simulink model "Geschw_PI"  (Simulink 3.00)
settings: Solver=ode5  SolverMode=SingleTasking  StartTime=0.0  StopTime=0.4  RelTol=1e-3  AbsTol=1e-6
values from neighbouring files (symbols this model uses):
  bm = 4    [PI_Par.m]    (also in Red_Par.m)
  K_St = 1/FD_Stern    (= 2.27848101266)    [PI_Par.m]    (also in Red_Par.m = 1/FD_Stern)
  KP = (1/K_St)*(2*d*T_St-T)/T    (= 23.3767988889)    [PI_Par.m]
  qA = 0    [PI_Par.m]    (also in Red_Par.m)
  T_St = M_Stern/FD_Stern    (= 2.82860759494)    [PI_Par.m]    (also in Red_Par.m = M_Stern/FD_Stern)
  tb = vm/bm    (= 0.5)    [PI_Par.m]    (also in Red_Par.m)
  te = tv+tb    (= 1.2853981634)    [PI_Par.m]    (also in Red_Par.m)
  TN = T*(2*d-T/T_St)    (= 0.0693971006366)    [PI_Par.m]
  tv = se/vm    (= 0.785398163397)    [PI_Par.m]    (also in Red_Par.m)
  Vorz = 1    [PI_Par.m]    (also in Red_Par.m)
  z0 = (1/KM)*(rh)    (= 1.25)    [PI_Par.m]    (also in Red_Par.m = (1/KM)*(rh))

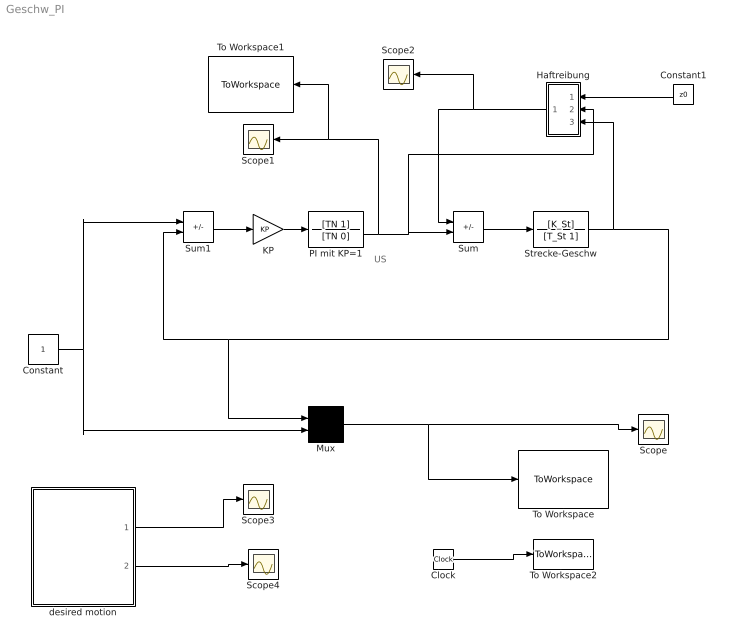
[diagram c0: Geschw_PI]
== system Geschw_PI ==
  note: US
  Clock : Clock
  Constant : Constant  Value=1
  Constant1 : Constant  Orientation=left  Value=z0
  Haftreibung : Subsystem  Orientation=left
  KP : Gain  Gain=KP  SaturateOnIntegerOverflow=on
  Mux : Mux  Inputs=2
  PI mit KP=1 : TransferFcn  Numerator=[TN 1]  Denominator=[TN 0]
  Scope{,1..4} (5 alike) : Scope
  Strecke-Geschw : TransferFcn  Numerator=[K_St]  Denominator=[T_St 1]
  Sum : Sum  Inputs=-+  SaturateOnIntegerOverflow=on
  Sum1 : Sum  Inputs=+-  SaturateOnIntegerOverflow=on
  To Workspace : ToWorkspace  VariableName=PI_MMin_SP  SampleTime=0.001  SaveFormat=Matrix
  To Workspace1 : ToWorkspace  VariableName=PI_MMin_US_SP  SampleTime=0.001  SaveFormat=Matrix
  To Workspace2 : ToWorkspace  VariableName=Zeit_SP  SampleTime=0.001  SaveFormat=Matrix
  desired motion : Subsystem
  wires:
  Sum1/1 -> KP/1
  KP/1 -> PI mit KP=1/1
  PI mit KP=1/1 -> Sum/2, Haftreibung/2(US), Scope1/1, To Workspace1/1
  Strecke-Geschw/1 -> Sum1/2, Mux/1, Haftreibung/3(qp)
  Sum/1 -> Strecke-Geschw/1
  Constant1/1 -> Haftreibung/1(z0)
  Haftreibung/1(Out1) -> Sum/1, Scope2/1
  Mux/1 -> Scope/1, To Workspace/1
  Clock/1 -> To Workspace2/1
  desired motion/1(qd) -> Scope3/1
  desired motion/2(vd) -> Scope4/1
  Constant/1 -> Mux/2, Sum1/1

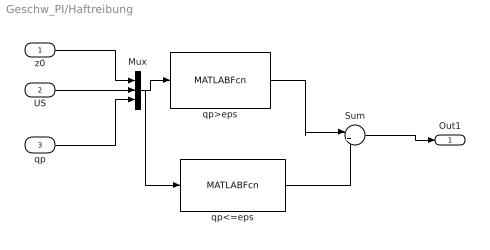
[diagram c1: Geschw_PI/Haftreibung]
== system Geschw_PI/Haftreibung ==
  z0 : Inport  Port=1  PortWidth=-1  SampleTime=-1  DataType=auto
  US : Inport  Port=2  PortWidth=-1  SampleTime=-1  DataType=auto
  qp : Inport  Port=3  PortWidth=-1  SampleTime=-1  DataType=auto
  Mux : Mux  Inputs=3
  Sum : Sum  Inputs=|++  SaturateOnIntegerOverflow=on
  qp<=eps : MATLABFcn  MATLABFcn=(abs(u(3)) < eps) *min(abs(u(2)),u(1))* sign(u(2))*sign(u(1))  OutputWidth=1  OutputSignalType=auto
  qp>eps : MATLABFcn  MATLABFcn=(abs(u(3)) > eps) * sign(u(3))*u(1)  OutputWidth=1  OutputSignalType=auto
  Out1 : Outport  Port=1  InitialOutput=0
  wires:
  z0/1 -> Mux/1
  US/1 -> Mux/2
  qp/1 -> Mux/3
  Mux/1 -> qp>eps/1, qp<=eps/1
  Sum/1 -> Out1/1
  qp>eps/1 -> Sum/1
  qp<=eps/1 -> Sum/2

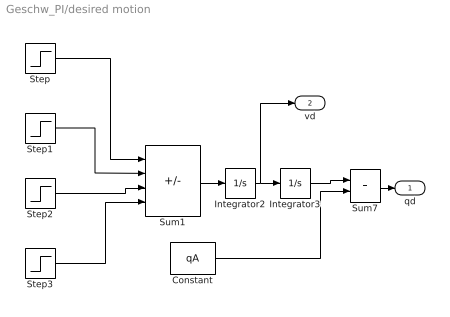
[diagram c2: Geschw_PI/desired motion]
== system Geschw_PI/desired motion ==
  Constant : Constant  Value=qA
  Integrator2 : Integrator  ExternalReset=none  InitialConditionSource=internal  InitialCondition=0  LimitOutput=off  UpperSaturationLimit=inf  LowerSaturationLimit=-inf  ShowSaturationPort=off  ShowStatePort=off  AbsoluteTolerance=auto
  Integrator3 : Integrator  ExternalReset=none  InitialConditionSource=internal  InitialCondition=0  LimitOutput=off  UpperSaturationLimit=inf  LowerSaturationLimit=-inf  ShowSaturationPort=off  ShowStatePort=off  AbsoluteTolerance=auto
  Step : Step  Time=0  Before=0  After=bm*Vorz  SampleTime=0.005
  Step1 : Step  Time=tb  Before=0  After=bm*Vorz  SampleTime=0.005
  Step2 : Step  Time=tv  Before=0  After=bm*Vorz  SampleTime=0.005
  Step3 : Step  Time=te  Before=0  After=bm*Vorz  SampleTime=0.005
  Sum1 : Sum  Inputs=+--+  SaturateOnIntegerOverflow=on
  Sum7 : Sum  Inputs=++  SaturateOnIntegerOverflow=on
  qd : Outport  Port=1  InitialOutput=0
  vd : Outport  Port=2
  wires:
  Step/1 -> Sum1/1
  Step1/1 -> Sum1/2
  Step2/1 -> Sum1/3
  Step3/1 -> Sum1/4
  Sum1/1 -> Integrator2/1
  Integrator2/1 -> Integrator3/1, vd/1
  Constant/1 -> Sum7/2
  Integrator3/1 -> Sum7/1
  Sum7/1 -> qd/1
